PROGRAM P_Prog5
VAR

	fbKL6401 					: FB_LON_KL6401;

	fbREAD_125		: FB_READ_125_SNVT_ph;
	fbSEND_125		: FB_SEND_125_SNVT_ph;

	fbREAD_126		: FB_READ_126_SNVT_ph_f;
	fbSEND_126		: FB_SEND_126_SNVT_ph_f;

	fbREAD_127		: FB_READ_127_SNVT_chlr_status;
	fbSEND_127		: FB_SEND_127_SNVT_chlr_status;

	fbREAD_128		: FB_READ_128_SNVT_tod_event;
	fbSEND_128		: FB_SEND_128_SNVT_tod_event;

	fbREAD_129		: FB_READ_129_SNVT_smo_obscur;
	fbSEND_129		: FB_SEND_129_SNVT_smo_obscur;

	fbREAD_130		: FB_READ_130_SNVT_fire_test;
	fbSEND_130		: FB_SEND_130_SNVT_fire_test;

	fbREAD_131		: FB_READ_131_SNVT_temp_ror;
	fbSEND_131		: FB_SEND_131_SNVT_temp_ror;

	fbREAD_132		: FB_READ_132_SNVT_fire_init;
	fbSEND_132		: FB_SEND_132_SNVT_fire_init;

	fbREAD_133		: FB_READ_133_SNVT_fire_indcte;
	fbSEND_133		: FB_SEND_133_SNVT_fire_indcte;

	fbREAD_134		: FB_READ_134_SNVT_time_zone;
	fbSEND_134		: FB_SEND_134_SNVT_time_zone;

	fbREAD_135		: FB_READ_135_SNVT_earth_pos;
	fbSEND_135		: FB_SEND_135_SNVT_earth_pos;

	fbREAD_136		: FB_READ_136_SNVT_reg_val;
	fbSEND_136		: FB_SEND_136_SNVT_reg_val;

	fbREAD_137		: FB_READ_137_SNVT_reg_val_ts;
	fbSEND_137		: FB_SEND_137_SNVT_reg_val_ts;

	fbREAD_138		: FB_READ_138_SNVT_volt_ac;
	fbSEND_138		: FB_SEND_138_SNVT_volt_ac;

	fbREAD_139		: FB_READ_139_SNVT_amp_ac;
	fbSEND_139		: FB_SEND_139_SNVT_amp_ac;

(*
	fbREAD_140		: FB_READ_109_SNVT_occupancy;
	fbSEND_140		: FB_SEND_109_SNVT_occupancy;

	fbREAD_141		: FB_READ_110_SNVT_area;
	fbSEND_141		: FB_SEND_110_SNVT_area;

	fbREAD_142		: FB_READ_111_SNVT_hvac_overid;
	fbSEND_142		: FB_SEND_111_SNVT_hvac_overid;
*)
	fbREAD_143		: FB_READ_143_SNVT_turbidity;
	fbSEND_143		: FB_SEND_143_SNVT_turbidity;

	fbREAD_144		: FB_READ_144_SNVT_turbidity_f;
	fbSEND_144		: FB_SEND_144_SNVT_turbidity_f;

	fbREAD_145		: FB_READ_145_SNVT_hvac_type;
	fbSEND_145		: FB_SEND_145_SNVT_hvac_type;

	fbREAD_146		: FB_READ_146_SNVT_elec_kwh_l;
	fbSEND_146		: FB_SEND_146_SNVT_elec_kwh_l;

	fbREAD_147		: FB_READ_147_SNVT_temp_diff_p;
	fbSEND_147		: FB_SEND_147_SNVT_temp_diff_p;

	fbREAD_148		: FB_READ_148_SNVT_ctrl_req;
	fbSEND_148		: FB_SEND_148_SNVT_ctrl_req;

	fbREAD_149		: FB_READ_149_SNVT_ctrl_resp;
	fbSEND_149		: FB_SEND_149_SNVT_ctrl_resp;

	fbREAD_150		: FB_READ_150_SNVT_ptz;
	fbSEND_150		: FB_SEND_150_SNVT_ptz;

	fbREAD_151		: FB_READ_151_SNVT_privacyzone;
	fbSEND_151		: FB_SEND_151_SNVT_privacyzone;

	fbREAD_152		: FB_READ_152_SNVT_pos_ctrl;
	fbSEND_152		: FB_SEND_152_SNVT_pos_ctrl;

	fbREAD_153		: FB_READ_153_SNVT_enthalpy;
	fbSEND_153		: FB_SEND_153_SNVT_enthalpy;

	fbREAD_154		: FB_READ_154_SNVT_gfci_status;
	fbSEND_154		: FB_SEND_154_SNVT_gfci_status;

	fbREAD_155		: FB_READ_155_SNVT_motor_state;
	fbSEND_155		: FB_SEND_155_SNVT_motor_state;

	fbREAD_156		: FB_READ_156_SNVT_pumpset_mn;
	fbSEND_156		: FB_SEND_156_SNVT_pumpset_mn;

	fbREAD_157		: FB_READ_157_SNVT_ex_control;
	fbSEND_157		: FB_SEND_157_SNVT_ex_control;

	fbREAD_158		: FB_READ_158_SNVT_pumpset_sn;
	fbSEND_158		: FB_SEND_158_SNVT_pumpset_sn;
END_VAR

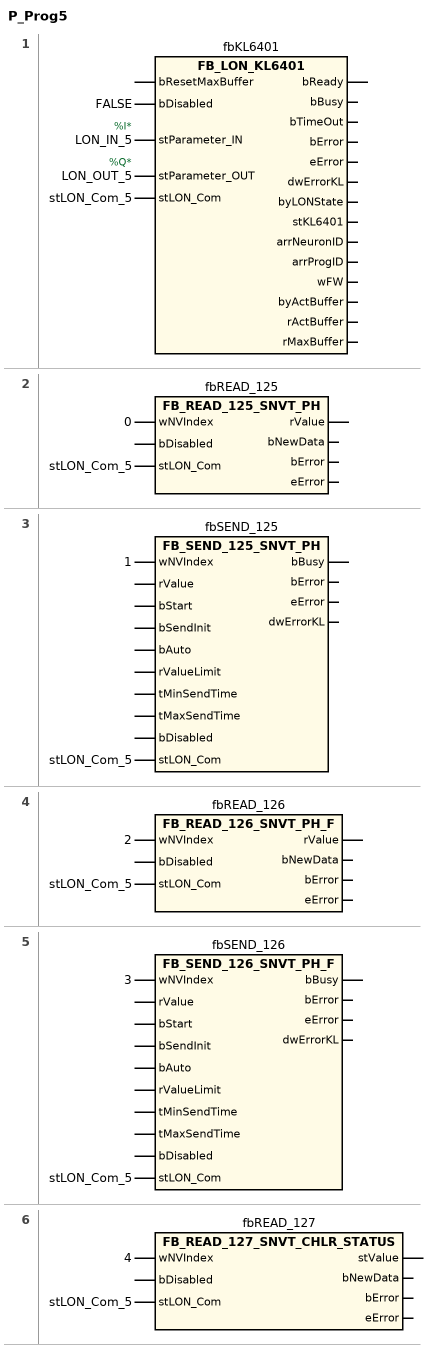
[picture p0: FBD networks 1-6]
// NETWORK 1
//   LON_IN_5: AT %I*
//   LON_OUT_5: AT %Q*
fbKL6401(
    bDisabled := FALSE,
    stParameter_IN := LON_IN_5,
    stParameter_OUT := LON_OUT_5,
    stLON_Com := stLON_Com_5); // FB_LON_KL6401

// NETWORK 2
fbREAD_125(wNVIndex := 0, stLON_Com := stLON_Com_5); // FB_READ_125_SNVT_PH

// NETWORK 3
fbSEND_125(wNVIndex := 1, stLON_Com := stLON_Com_5); // FB_SEND_125_SNVT_PH

// NETWORK 4
fbREAD_126(wNVIndex := 2, stLON_Com := stLON_Com_5); // FB_READ_126_SNVT_PH_F

// NETWORK 5
fbSEND_126(wNVIndex := 3, stLON_Com := stLON_Com_5); // FB_SEND_126_SNVT_PH_F

// NETWORK 6
fbREAD_127(wNVIndex := 4, stLON_Com := stLON_Com_5); // FB_READ_127_SNVT_CHLR_STATUS

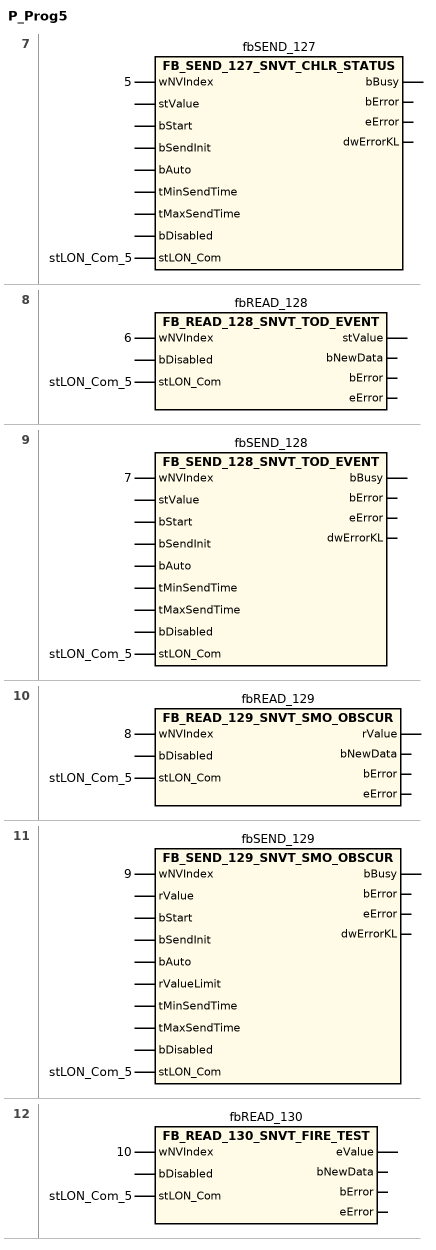
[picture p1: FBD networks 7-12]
// NETWORK 7
fbSEND_127(wNVIndex := 5, stLON_Com := stLON_Com_5); // FB_SEND_127_SNVT_CHLR_STATUS

// NETWORK 8
fbREAD_128(wNVIndex := 6, stLON_Com := stLON_Com_5); // FB_READ_128_SNVT_TOD_EVENT

// NETWORK 9
fbSEND_128(wNVIndex := 7, stLON_Com := stLON_Com_5); // FB_SEND_128_SNVT_TOD_EVENT

// NETWORK 10
fbREAD_129(wNVIndex := 8, stLON_Com := stLON_Com_5); // FB_READ_129_SNVT_SMO_OBSCUR

// NETWORK 11
fbSEND_129(wNVIndex := 9, stLON_Com := stLON_Com_5); // FB_SEND_129_SNVT_SMO_OBSCUR

// NETWORK 12
fbREAD_130(wNVIndex := 10, stLON_Com := stLON_Com_5); // FB_READ_130_SNVT_FIRE_TEST

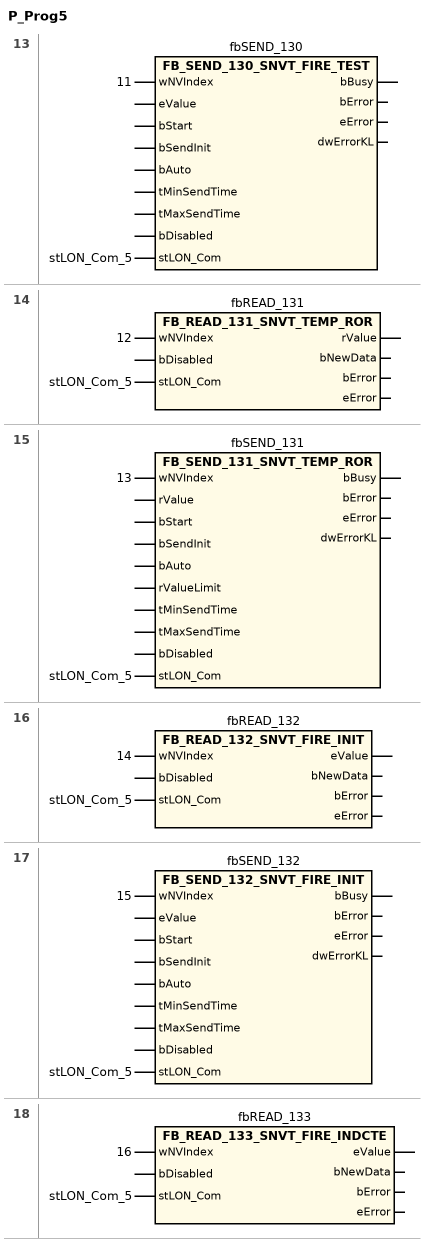
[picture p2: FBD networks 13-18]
// NETWORK 13
fbSEND_130(wNVIndex := 11, stLON_Com := stLON_Com_5); // FB_SEND_130_SNVT_FIRE_TEST

// NETWORK 14
fbREAD_131(wNVIndex := 12, stLON_Com := stLON_Com_5); // FB_READ_131_SNVT_TEMP_ROR

// NETWORK 15
fbSEND_131(wNVIndex := 13, stLON_Com := stLON_Com_5); // FB_SEND_131_SNVT_TEMP_ROR

// NETWORK 16
fbREAD_132(wNVIndex := 14, stLON_Com := stLON_Com_5); // FB_READ_132_SNVT_FIRE_INIT

// NETWORK 17
fbSEND_132(wNVIndex := 15, stLON_Com := stLON_Com_5); // FB_SEND_132_SNVT_FIRE_INIT

// NETWORK 18
fbREAD_133(wNVIndex := 16, stLON_Com := stLON_Com_5); // FB_READ_133_SNVT_FIRE_INDCTE

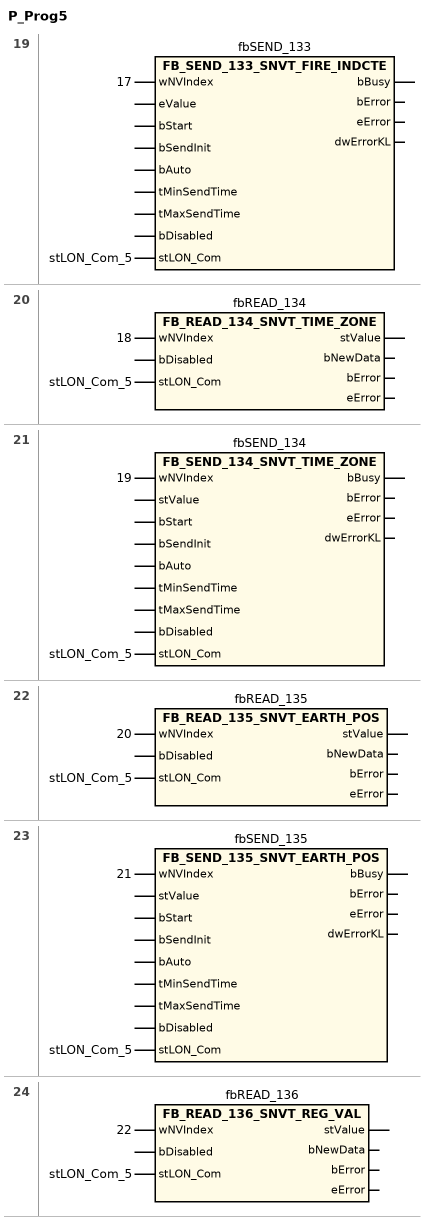
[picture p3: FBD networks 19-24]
// NETWORK 19
fbSEND_133(wNVIndex := 17, stLON_Com := stLON_Com_5); // FB_SEND_133_SNVT_FIRE_INDCTE

// NETWORK 20
fbREAD_134(wNVIndex := 18, stLON_Com := stLON_Com_5); // FB_READ_134_SNVT_TIME_ZONE

// NETWORK 21
fbSEND_134(wNVIndex := 19, stLON_Com := stLON_Com_5); // FB_SEND_134_SNVT_TIME_ZONE

// NETWORK 22
fbREAD_135(wNVIndex := 20, stLON_Com := stLON_Com_5); // FB_READ_135_SNVT_EARTH_POS

// NETWORK 23
fbSEND_135(wNVIndex := 21, stLON_Com := stLON_Com_5); // FB_SEND_135_SNVT_EARTH_POS

// NETWORK 24
fbREAD_136(wNVIndex := 22, stLON_Com := stLON_Com_5); // FB_READ_136_SNVT_REG_VAL

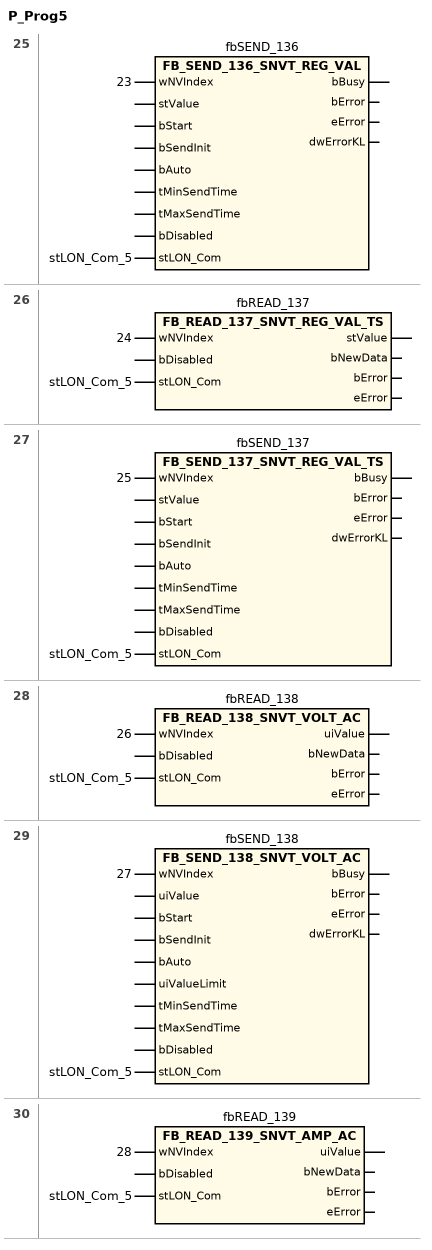
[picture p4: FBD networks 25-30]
// NETWORK 25
fbSEND_136(wNVIndex := 23, stLON_Com := stLON_Com_5); // FB_SEND_136_SNVT_REG_VAL

// NETWORK 26
fbREAD_137(wNVIndex := 24, stLON_Com := stLON_Com_5); // FB_READ_137_SNVT_REG_VAL_TS

// NETWORK 27
fbSEND_137(wNVIndex := 25, stLON_Com := stLON_Com_5); // FB_SEND_137_SNVT_REG_VAL_TS

// NETWORK 28
fbREAD_138(wNVIndex := 26, stLON_Com := stLON_Com_5); // FB_READ_138_SNVT_VOLT_AC

// NETWORK 29
fbSEND_138(wNVIndex := 27, stLON_Com := stLON_Com_5); // FB_SEND_138_SNVT_VOLT_AC

// NETWORK 30
fbREAD_139(wNVIndex := 28, stLON_Com := stLON_Com_5); // FB_READ_139_SNVT_AMP_AC

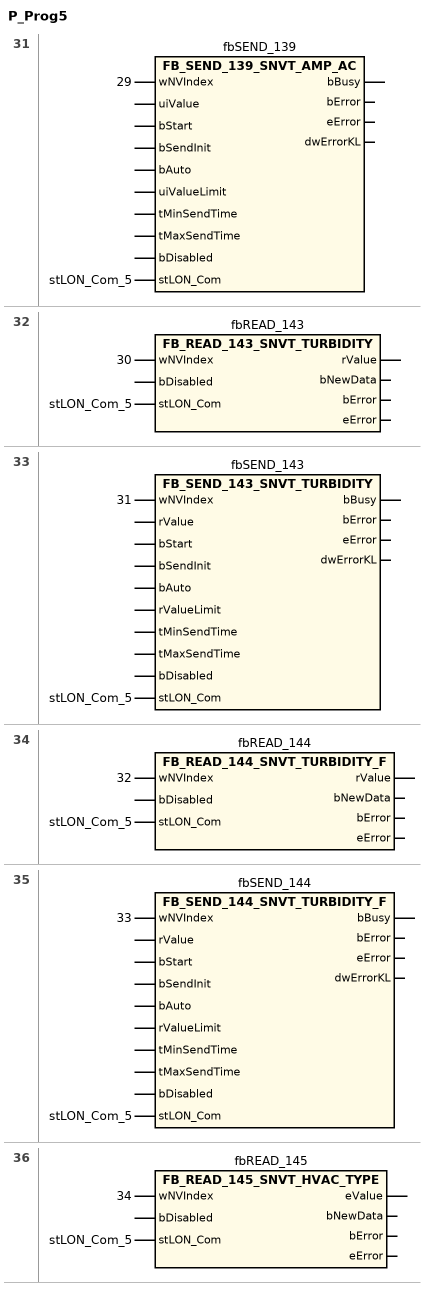
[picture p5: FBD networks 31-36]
// NETWORK 31
fbSEND_139(wNVIndex := 29, stLON_Com := stLON_Com_5); // FB_SEND_139_SNVT_AMP_AC

// NETWORK 32
//   fbREAD_143: fbREAD_140 : FB_READ_109_SNVT_occupancy; fbSEND_140 : FB_SEND_109_SNVT_occupancy; fbREAD_141 : FB_READ_110_SNVT_area; fbSEND_141 : FB_SEND_110_SNVT_area; fbREAD_142 : FB_READ_111_SNVT_hvac_overid; fbSEND_142 : FB_SEND_111_SNVT_hvac_overid;
fbREAD_143(wNVIndex := 30, stLON_Com := stLON_Com_5); // FB_READ_143_SNVT_TURBIDITY

// NETWORK 33
fbSEND_143(wNVIndex := 31, stLON_Com := stLON_Com_5); // FB_SEND_143_SNVT_TURBIDITY

// NETWORK 34
fbREAD_144(wNVIndex := 32, stLON_Com := stLON_Com_5); // FB_READ_144_SNVT_TURBIDITY_F

// NETWORK 35
fbSEND_144(wNVIndex := 33, stLON_Com := stLON_Com_5); // FB_SEND_144_SNVT_TURBIDITY_F

// NETWORK 36
fbREAD_145(wNVIndex := 34, stLON_Com := stLON_Com_5); // FB_READ_145_SNVT_HVAC_TYPE

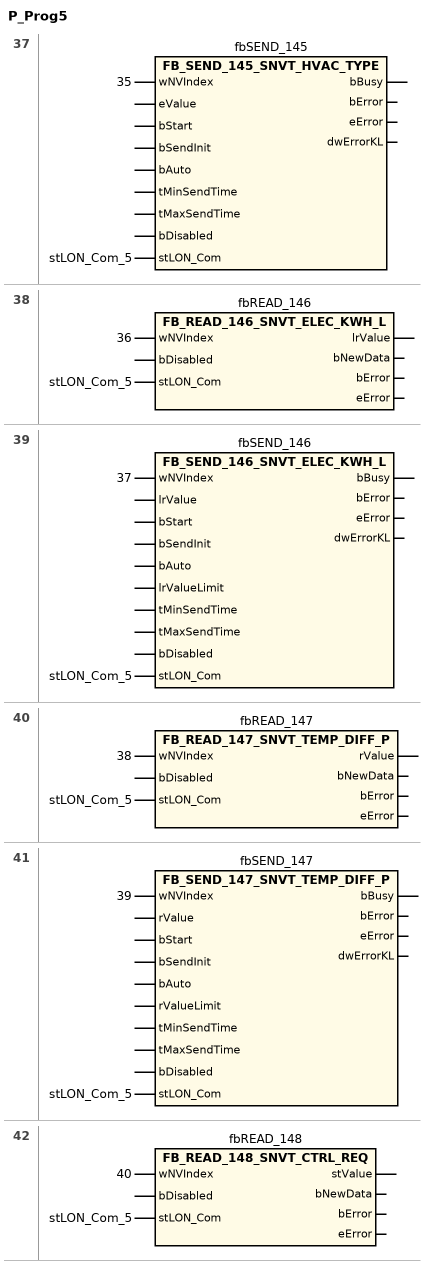
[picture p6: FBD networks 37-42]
// NETWORK 37
fbSEND_145(wNVIndex := 35, stLON_Com := stLON_Com_5); // FB_SEND_145_SNVT_HVAC_TYPE

// NETWORK 38
fbREAD_146(wNVIndex := 36, stLON_Com := stLON_Com_5); // FB_READ_146_SNVT_ELEC_KWH_L

// NETWORK 39
fbSEND_146(wNVIndex := 37, stLON_Com := stLON_Com_5); // FB_SEND_146_SNVT_ELEC_KWH_L

// NETWORK 40
fbREAD_147(wNVIndex := 38, stLON_Com := stLON_Com_5); // FB_READ_147_SNVT_TEMP_DIFF_P

// NETWORK 41
fbSEND_147(wNVIndex := 39, stLON_Com := stLON_Com_5); // FB_SEND_147_SNVT_TEMP_DIFF_P

// NETWORK 42
fbREAD_148(wNVIndex := 40, stLON_Com := stLON_Com_5); // FB_READ_148_SNVT_CTRL_REQ

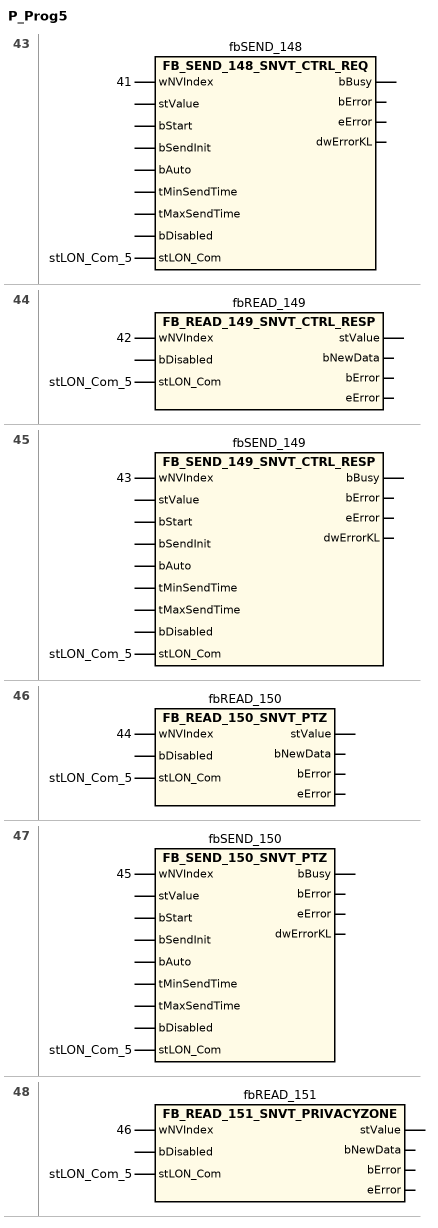
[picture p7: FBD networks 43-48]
// NETWORK 43
fbSEND_148(wNVIndex := 41, stLON_Com := stLON_Com_5); // FB_SEND_148_SNVT_CTRL_REQ

// NETWORK 44
fbREAD_149(wNVIndex := 42, stLON_Com := stLON_Com_5); // FB_READ_149_SNVT_CTRL_RESP

// NETWORK 45
fbSEND_149(wNVIndex := 43, stLON_Com := stLON_Com_5); // FB_SEND_149_SNVT_CTRL_RESP

// NETWORK 46
fbREAD_150(wNVIndex := 44, stLON_Com := stLON_Com_5); // FB_READ_150_SNVT_PTZ

// NETWORK 47
fbSEND_150(wNVIndex := 45, stLON_Com := stLON_Com_5); // FB_SEND_150_SNVT_PTZ

// NETWORK 48
fbREAD_151(wNVIndex := 46, stLON_Com := stLON_Com_5); // FB_READ_151_SNVT_PRIVACYZONE

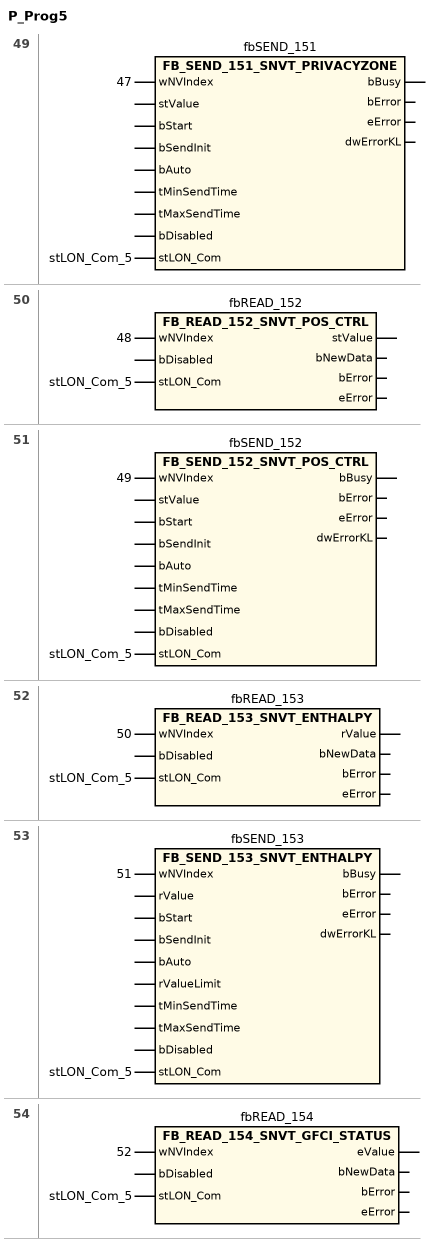
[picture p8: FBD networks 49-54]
// NETWORK 49
fbSEND_151(wNVIndex := 47, stLON_Com := stLON_Com_5); // FB_SEND_151_SNVT_PRIVACYZONE

// NETWORK 50
fbREAD_152(wNVIndex := 48, stLON_Com := stLON_Com_5); // FB_READ_152_SNVT_POS_CTRL

// NETWORK 51
fbSEND_152(wNVIndex := 49, stLON_Com := stLON_Com_5); // FB_SEND_152_SNVT_POS_CTRL

// NETWORK 52
fbREAD_153(wNVIndex := 50, stLON_Com := stLON_Com_5); // FB_READ_153_SNVT_ENTHALPY

// NETWORK 53
fbSEND_153(wNVIndex := 51, stLON_Com := stLON_Com_5); // FB_SEND_153_SNVT_ENTHALPY

// NETWORK 54
fbREAD_154(wNVIndex := 52, stLON_Com := stLON_Com_5); // FB_READ_154_SNVT_GFCI_STATUS

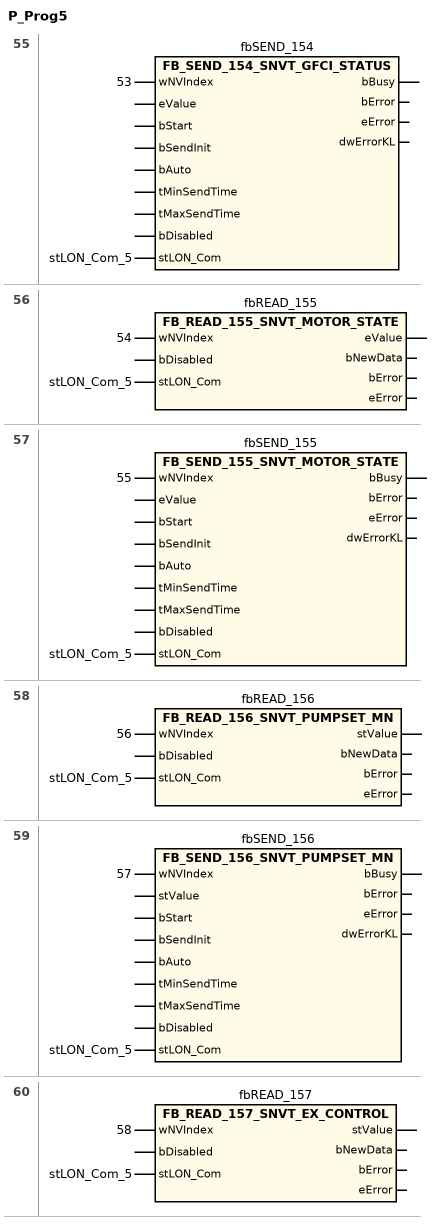
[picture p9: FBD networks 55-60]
// NETWORK 55
fbSEND_154(wNVIndex := 53, stLON_Com := stLON_Com_5); // FB_SEND_154_SNVT_GFCI_STATUS

// NETWORK 56
fbREAD_155(wNVIndex := 54, stLON_Com := stLON_Com_5); // FB_READ_155_SNVT_MOTOR_STATE

// NETWORK 57
fbSEND_155(wNVIndex := 55, stLON_Com := stLON_Com_5); // FB_SEND_155_SNVT_MOTOR_STATE

// NETWORK 58
fbREAD_156(wNVIndex := 56, stLON_Com := stLON_Com_5); // FB_READ_156_SNVT_PUMPSET_MN

// NETWORK 59
fbSEND_156(wNVIndex := 57, stLON_Com := stLON_Com_5); // FB_SEND_156_SNVT_PUMPSET_MN

// NETWORK 60
fbREAD_157(wNVIndex := 58, stLON_Com := stLON_Com_5); // FB_READ_157_SNVT_EX_CONTROL

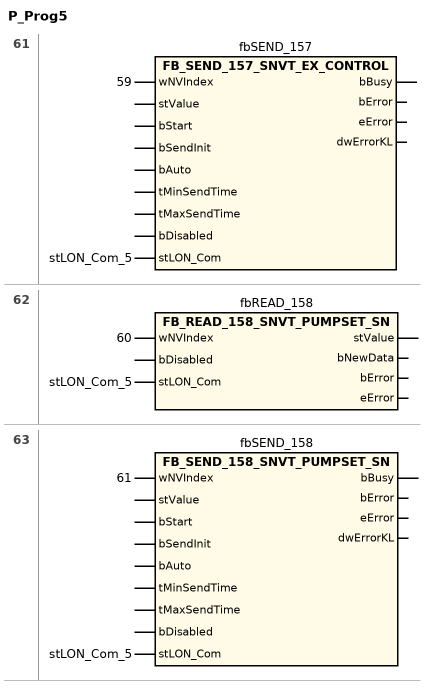
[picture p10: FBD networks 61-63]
// NETWORK 61
fbSEND_157(wNVIndex := 59, stLON_Com := stLON_Com_5); // FB_SEND_157_SNVT_EX_CONTROL

// NETWORK 62
fbREAD_158(wNVIndex := 60, stLON_Com := stLON_Com_5); // FB_READ_158_SNVT_PUMPSET_SN

// NETWORK 63
fbSEND_158(wNVIndex := 61, stLON_Com := stLON_Com_5); // FB_SEND_158_SNVT_PUMPSET_SN

END_PROGRAM
